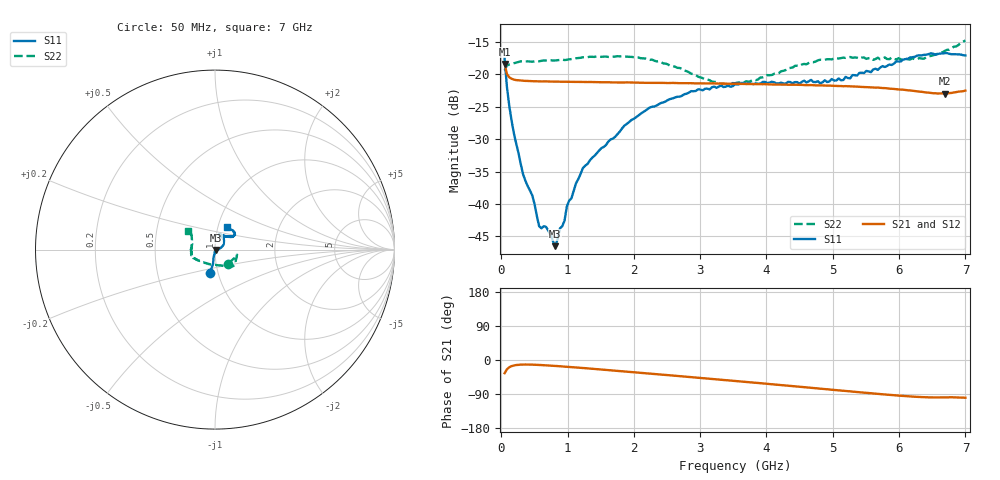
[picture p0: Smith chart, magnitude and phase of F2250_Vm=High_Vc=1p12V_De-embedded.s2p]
! Integrated Device Technology
! Corporate Headquarters
! 6024 Silver Creek Valley Road
! San Jose, CA 95138  USA
! Phone:  1-408-284-8200
! Toll Free:  1-800-223-1366
! Webpage:  http://www.idt.com/
! Timing and RF Division
! 515 Groton Road, Suite 102
! Westford, MA 01886-6024
! Device:  F2250
! Description: Voltage Variable RF Attenuator
! Frequency:  50.0 -  6000.00 MHz
! Package:  3x3 mm Thin QFN Plastic Package: 16 pin
! Ports:  2 RF, 3 DC
!  Pin  1  = GND
!  Pin  2  = NC
!  Pin  3  = RF1  = Port 1
!  Pin  4  = NC
!  Pin  5  = GND
!  Pin  6  = GND
!  Pin  7  = GND
!  Pin  8  = GND
!  Pin  9  = NC
!  Pin 10  = RF2  = Port 2
!  Pin 11  = NC
!  Pin 12  = GND
!  Pin 13  = GND
!  Pin 14  = VCNTRL
!  Pin 15  = VDD
!  Pin 16  = VMODE
! Vcntrl:  1.120 Volts
! Vmode:  +3.300 Volts
! Vdd:  +3.30  Volts
! Current:  1.329 mA
! Data:  The device was measured on a the F2250 evaluation board which has
!  individual transmission lines to the RF pins.  Data was collected
!  using a calibrated network analyzer.  The evaluation board was
!  de-embedded using a TRL calibration technique.
!  The reference plane is the edge of the package pin.
! Misc:  SN 10
!  Action Tracker AT0258
! Date Measured:  2014-11-26
! Date:  2015-10-15  MJV
! Note:
!  Integrated Device Technology supplies this data as a sample of measured
!  data at the package pin for this product.  Your particular data for this
!  product may vary.
!  Data was taken at 25 degrees C.
!  Integrated Device Technology reserves the right to change this data at anytime.
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# GHz S dB R 50
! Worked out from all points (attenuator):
!   201 points, 50 MHz to 7 GHz, reference 50 ohm
!   highest |S21| = -18.37 dB at 50 MHz (marker M1); lowest = -22.9 dB at 6.687 GHz (marker M2)
!   lowest |S11| = -46.5 dB at 814.5 MHz (marker M3), VSWR 1.01, Z = 50.4 - j0.21 ohm
!   |S11| at or under -10 dB: start of sweep to end of sweep
!   |S22| runs from -21.5 to -14.8 dB; largest |S21 - S12| = 0.00037
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0.05  -17.53 -102.3  -18.37 -34.8  -18.38 -34.8  -19.39 -46.4
0.08475  -21.90 -97.9  -19.91 -24.6  -19.90 -24.5  -18.61 -23.7
0.15425  -27.04 -100.4  -20.66 -16.2  -20.66 -16.2  -18.41 -14.4
0.328  -35.39 -95.5  -20.97 -12.0  -20.97 -12.0  -17.96 -12.9
0.467  -38.65 -94.2  -21.03 -12.3  -21.03 -12.3  -18.03 -14.8
0.57125  -43.44 -74.5  -21.06 -13.1  -21.08 -13.1  -17.96 -17.3
0.6755  -43.53 -64.6  -21.07 -14.1  -21.07 -14.1  -17.85 -19.3
0.8145  -46.50 -26.1  -21.10 -15.7  -21.11 -15.7  -17.84 -23.0
0.884  -43.76 -19.8  -21.12 -16.5  -21.12 -16.5  -17.75 -25.1
0.9535  -42.57 -27.0  -21.13 -17.4  -21.13 -17.4  -17.78 -26.3
0.98825  -40.40 -21.1  -21.15 -17.8  -21.16 -17.8  -17.74 -27.0
1.2315  -34.44 1.6  -21.16 -21.1  -21.16 -21.1  -17.34 -31.7
1.857  -27.89 21.2  -21.24 -30.1  -21.23 -30.2  -17.21 -40.8
2.37825  -24.57 34.0  -21.29 -37.9  -21.29 -37.9  -17.95 -48.9
3.1775  -21.97 55.5  -21.38 -50.1  -21.38 -50.1  -21.11 -79.2
3.525  -21.53 65.6  -21.45 -55.4  -21.45 -55.4  -21.35 -103.7
4.7065  -21.16 69.0  -21.66 -73.9  -21.67 -73.9  -18.11 -156.5
5.15825  -20.86 52.7  -21.82 -81.1  -21.80 -81.1  -17.39 -165.3
5.85325  -18.46 37.4  -22.19 -91.9  -22.18 -92.1  -17.64 179.8
6.3745  -16.97 38.8  -22.73 -98.2  -22.73 -98.2  -17.58 161.7
6.68725  -16.70 46.2  -22.95 -98.6  -22.95 -98.7  -16.37 149.0
7  -17.06 61.9  -22.49 -99.5  -22.48 -99.8  -14.75 145.0
